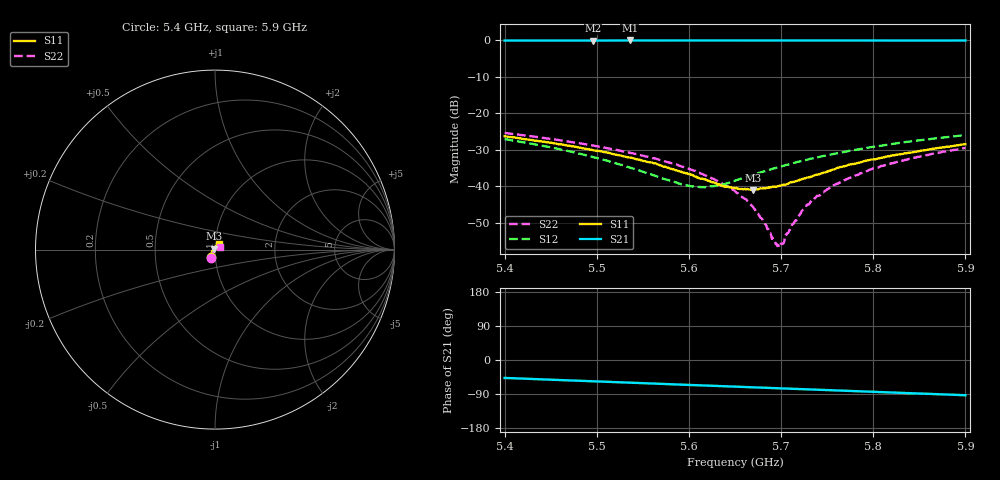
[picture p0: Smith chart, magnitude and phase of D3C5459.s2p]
! 11/4/2020 2:20:34 PM
! C:\USERS\DITOM\DESKTOP\SINGLE JUNCTION ISOLATOR DATA\5.4-5.9 GHZ (D3I5459).S2P
! CHANNEL.1
! TR.MEASUREMENT
! CORRECTED.DATA
# GHZ S RI R 50.0
! FREQ.GHZ  S11RE  S11IM  S21RE  S21IM  S12RE  S12IM  S22RE  S22IM
!; PortSelection: Port_12
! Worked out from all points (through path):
!   601 points, 5.4 GHz to 5.9 GHz, reference 50 ohm
!   highest |S21| = -0.06 dB at 5.536 GHz (marker M1); lowest = -0.1 dB at 5.496 GHz (marker M2)
!   lowest |S11| = -41.1 dB at 5.669 GHz (marker M3), VSWR 1.02, Z = 49.3 + j0.536 ohm
!   |S11| at or under -10 dB: start of sweep to end of sweep
!   |S22| runs from -56.4 to -25.4 dB; largest |S21 - S12| = 1
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5.4  -0.0247 -0.0417  0.6697 -0.7302  -0.0437 -0.0063  -0.0208 -0.0495
5.484167  -0.0213 -0.0255  0.5671 -0.8113  -0.027 0.00471  -0.0175 -0.034
5.495833  -0.0207 -0.0235  0.5518 -0.8212  -0.0244 0.00587  -0.0167 -0.032
5.535833  -0.019 -0.0159  0.5009 -0.8572  -0.0159 0.00843  -0.0143 -0.025
5.566667  -0.0164 -0.0109  0.4554 -0.8814  -0.0094 0.00956  -0.0119 -0.02
5.594167  -0.0141 -0.0062  0.4165 -0.901  -0.00342 0.00986  -0.00967 -0.0157
5.611667  -0.0124 -0.00342  0.3913 -0.9109  0.000212 0.00976  -0.00797 -0.013
5.636667  -0.01 0.000674  0.3543 -0.9257  0.00537 0.00918  -0.00551 -0.00916
5.65  -0.00899 0.00281  0.3356 -0.9336  0.00806 0.00872  -0.00423 -0.0074
5.6625  -0.00794 0.00457  0.3173 -0.9402  0.0106 0.00815  -0.00311 -0.00579
5.669167  -0.00699 0.00544  0.3076 -0.9434  0.0121 0.0076  -0.00215 -0.00485
5.681667  -0.00589 0.00724  0.2888 -0.949  0.0144 0.00712  -0.000773 -0.00312
5.6925  -0.00476 0.00867  0.2714 -0.9539  0.0165 0.00624  0.000529 -0.00177
5.698333  -0.00408 0.0093  0.2621 -0.957  0.0175 0.00565  0.00112 -0.00119
5.701667  -0.00384 0.00971  0.2568 -0.9584  0.0181 0.00553  0.00151 -0.000623
5.706667  -0.00309 0.0103  0.2493 -0.9606  0.019 0.00509  0.00228 3.17e-05
5.720833  -0.00125 0.0123  0.2283 -0.9658  0.0216 0.0039  0.00388 0.00165
5.734167  0.000593 0.0138  0.2076 -0.9703  0.0239 0.00247  0.00573 0.00331
5.755  0.00323 0.0164  0.175 -0.976  0.0275 0.000198  0.00821 0.00545
5.7675  0.00486 0.018  0.1554 -0.9796  0.0293 -0.00126  0.00982 0.00689
5.816667  0.0112 0.0231  0.0787 -0.9873  0.0363 -0.00808  0.0167 0.011
5.9  0.0235 0.0294  -0.0519 -0.99  0.0452 -0.0222  0.0291 0.0163
